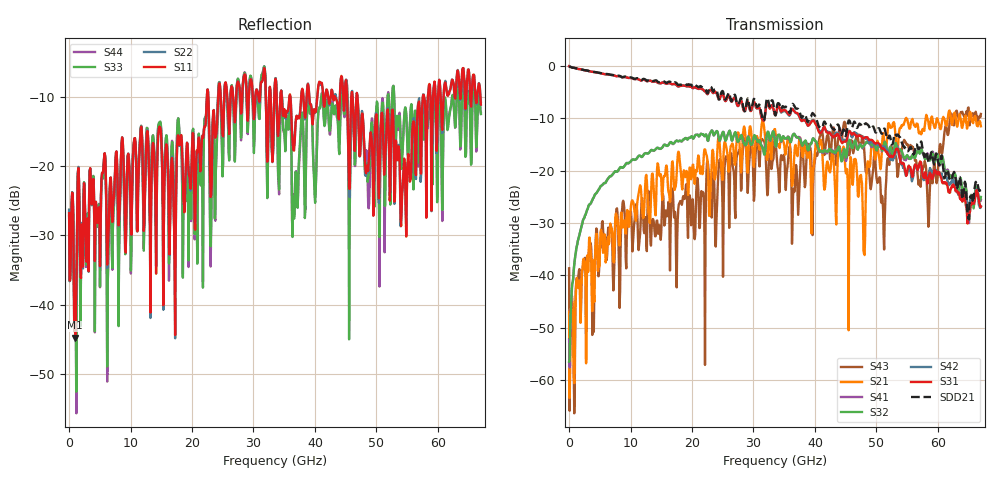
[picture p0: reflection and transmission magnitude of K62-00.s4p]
!Agilent Technologies,N5247A,US50470101,A.10.25.02
!Agilent N5247A: A.10.25.02
!Date: Tuesday, May 12, 2015 13:34:00
!Correction: Sdd11(Full 4 Port(1,2,3,4))
!Sdc11(Full 4 Port(1,2,3,4))
!Sdd12(Full 4 Port(1,2,3,4))
!Sdc12(Full 4 Port(1,2,3,4))
!Scd11(Full 4 Port(1,2,3,4))
!Scc11(Full 4 Port(1,2,3,4))
!Scd12(Full 4 Port(1,2,3,4))
!Scc12(Full 4 Port(1,2,3,4))
!Sdd21(Full 4 Port(1,2,3,4))
!Sdc21(Full 4 Port(1,2,3,4))
!Sdd22(Full 4 Port(1,2,3,4))
!Sdc22(Full 4 Port(1,2,3,4))
!Scd21(Full 4 Port(1,2,3,4))
!Scc21(Full 4 Port(1,2,3,4))
!Scd22(Full 4 Port(1,2,3,4))
!Scc22(Full 4 Port(1,2,3,4))
!Balanced Topology: BBAL
!S4P File: Measurements: <Sdd11,Sdc11,Sdd12,Sdc12>,
!<Scd11,Scc11,Scd12,Scc12>,
!<Sdd21,Sdc21,Sdd22,Sdc22>,
!<Scd21,Scc21,Scd22,Scc22>:
# Hz S  dB  R 50
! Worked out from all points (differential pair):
!   801 points, 10 MHz to 67 GHz, reference 50 ohm
!   strongest paths, dB at 10 MHz, 16.76 GHz, 33.51 GHz, 50.25 GHz, 67 GHz:
!     S31: 0.0, -3.5, -9.3, -14.7, -26.9
!     S42: 0.0, -3.5, -9.4, -15.0, -26.8
!     S32: -56.5, -14.7, -14.6, -15.5, -25.0
!     S41: -52.3, -14.8, -14.6, -15.5, -25.6
!     S21: -47.0, -18.4, -12.0, -14.9, -11.5
!     S43: -38.7, -23.4, -13.9, -22.2, -9.2
!   taken as a pair (ports 1,2 in; 3,4 out), SDD21 dB: 0.0, -3.3, -9.3, -12.0, -24.3
!   lowest |S11| = -44.8 dB at 1.015 GHz (marker M1), VSWR 1.01, Z = 50.6 + j0.124 ohm
!   |S11| at or under -10 dB: start of sweep to 22.43 GHz; 36.01 GHz to 37.77 GHz (1.759 GHz wide, 4.77 % of centre); 46.92 GHz to 57.58 GHz (10.66 GHz wide, 20.4 % of centre)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
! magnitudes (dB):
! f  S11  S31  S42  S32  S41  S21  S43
! 10 MHz  -26.8  0.0  0.0  -56.5  -52.3  -47.0  -38.7
! 1.015 GHz  -44.8  -0.4  -0.4  -36.3  -36.3  -46.7  -46.9
! 8.802 GHz  -17.7  -2.1  -2.1  -19.3  -19.4  -30.5  -25.7
! 17.85 GHz  -16.3  -3.9  -3.9  -14.4  -14.3  -16.4  -26.5
! 47.99 GHz  -16.5  -13.8  -13.7  -15.2  -15.2  -35.8  -15.5
! 52.18 GHz  -25.0  -17.4  -17.5  -15.5  -15.7  -11.4  -17.9
! 67 GHz  -11.2  -26.9  -26.8  -25.0  -25.6  -11.5  -9.2
